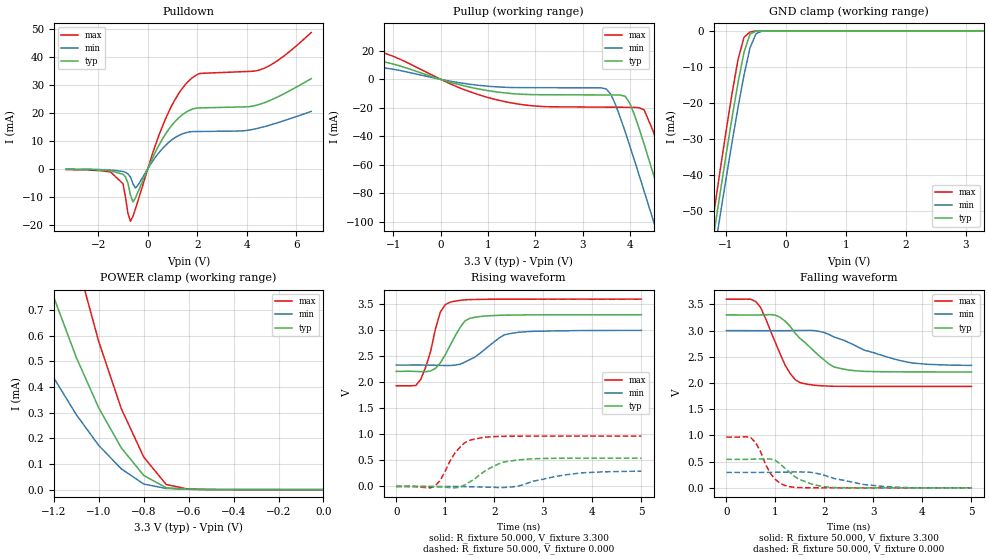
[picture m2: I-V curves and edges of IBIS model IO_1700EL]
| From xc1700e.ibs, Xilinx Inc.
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|   Model IO_1700EL
[Model]   IO_1700EL
Model_type   I/O
Polarity   Non-Inverting
Enable   Active-High
Vinl =   0.800V
Vinh =   2.000V
Vmeas =   1.650V
Cref =  50.000pF
Rref =   1.000M
Vref =  0.000V
C_comp   2.500pF   2.000pF   3.000pF
[Temperature Range]   50.000   100.000   0.000
[Voltage Range]   3.300V   3.000V   3.600V
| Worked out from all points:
|   slope of the pulldown table from 0 to 0.495 V, typ, clamps not added: 54.3 ohm
|   slope of the pullup table from 0 to 0.495 V, typ, clamps not added: 108 ohm
|   GND clamp passes 1 mA (typ) near -0.60 V on its own axis
|   POWER clamp passes 1 mA (typ) near -1.29 V on its own axis
|   rising waveform, R_fixture 50.000, V_fixture 3.300: 20-80 % time 389ps typ, 556ps min, 284ps max; typ from 2.21 V to 3.3 V
|   rising waveform, R_fixture 50.000, V_fixture 0.000: 20-80 % time 555ps typ, 874ps min, 383ps max; typ from 0 V to 0.543 V
|   falling waveform, R_fixture 50.000, V_fixture 3.300: 20-80 % time 706ps typ, 1.15ns min, 464ps max; typ from 3.3 V to 2.21 V
|   falling waveform, R_fixture 50.000, V_fixture 0.000: 20-80 % time 514ps typ, 842ps min, 321ps max; typ from 0.543 V to 0 V
[Pulldown]
| voltage   I(typ)   I(min)   I(max)
-3.3V     -200uA     -100uA     -300uA
-1.5V     -700uA     -440uA     -1.16mA
-1V       -1.96mA    -970uA     -5.37mA
-800mV    -5.18mA    -1.82mA    -15.96mA
-700mV    -9.413mA   -2.98mA    -18.75mA
-600mV    -11.79mA   -5.361mA   -17mA
-500mV    -10.41mA   -6.905mA   -14.34mA
600mV     10.73mA    7.28mA     15.37mA
1.6V      20.47mA    13.01mA    30.87mA
2.1V      21.72mA    13.3mA     34.02mA
4.7V      23.55mA    15.01mA    35.86mA
6.6V      32.17mA    20.46mA    48.6mA
[Pullup]
| voltage   I(typ)   I(min)   I(max)
-3.3V     22.13mA    12.6mA     35.43mA
-1.5V     14.78mA    9.662mA    22.26mA
1.2V      -8.899mA   -5.297mA   -14.5mA
3.5V      -10.96mA   -6.739mA   -19.54mA
3.7V      -10.99mA   -18.23mA   -19.58mA
4V        -16.93mA   -47.12mA   -19.65mA
4.3V      -45.58mA   -78.7mA    -21.49mA
4.5V      -67.23mA   -100mA     -37.14mA
4.7V      -89.56mA   -122mA     -58.71mA
4.9V      -112mA     -144mA     -81.58mA
5.1V      -135mA     -167mA     -105mA
6.6V      -313mA     -337mA     -289mA
[GND_clamp]
| voltage   I(typ)   I(min)   I(max)
-3.3V     -301mA     -296mA     -307mA
-1.3V     -67.23mA   -72.67mA   -61.75mA
-1.2V     -56.13mA   -62mA      -50.22mA
-1.1V     -45.21mA   -51.47mA   -38.91mA
-1V       -34.51mA   -41.11mA   -27.9mA
-900mV    -24.15mA   -31mA      -17.39mA
-800mV    -14.38mA   -21.28mA   -7.958mA
-700mV    -5.907mA   -12.25mA   -1.783mA
-600mV    -925uA     -4.729mA   -328uA
-500mV    -63.77uA   -772uA     -21.5uA
-400mV    -3.027uA   -71.54uA   -1.321uA
3.3V      152pA      11.15nA    59.2pA
[POWER_clamp]
| voltage   I(typ)   I(min)   I(max)
-3.3V     9.547mA    5.776mA    15.34mA
-1.4V     1.31mA     780uA      2.172mA
-1.3V     1.015mA    598uA      1.703mA
-1.2V     749uA      435uA      1.276mA
-1.1V     515uA      292uA      898uA
-1V       318uA      172uA      576uA
-900mV    163uA      81.04uA    316uA
-800mV    55.24uA    21.71uA    127uA
-700mV    7.221uA    4.5uA      19.75uA
-600mV    1.258uA    1.103uA    1.726uA
0V        152pA      1.498nA    69.06pA
[Ramp]
| variable   typ   min   max
dV/dt_r   0.326/0.560n   0.175/0.857n   0.581/0.376n
dV/dt_f   0.653/0.707n   0.398/1.106n   0.999/0.456n
R_load = 50.000
[Rising Waveform]
R_fixture = 50.000
V_fixture = 3.300
V_fixture_min = 3.000
V_fixture_max = 3.600
L_fixture = 0.000H
C_fixture = 0.000F
| time   V(typ)   V(min)   V(max)
0s        2.212V     2.333V     1.935V
400ps     2.21V      2.334V     1.94V
500ps     2.206V     2.334V     2.056V
700ps     2.218V     2.332V     2.589V
900ps     2.375V     2.327V     3.35V
1.1ns     2.711V     2.324V     3.541V
1.4ns     3.179V     2.389V     3.586V
1.6ns     3.251V     2.483V     3.593V
2.3ns     3.293V     2.934V     3.599V
5ns       3.3V       2.999V     3.6V
[Rising Waveform]
R_fixture = 50.000
V_fixture = 0.000
V_fixture_min = 0.000
V_fixture_max = 0.000
L_fixture = 0.000H
C_fixture = 0.000F
| time   V(typ)   V(min)   V(max)
0s        0V         0V         0V
800ps     -6.525mV   342uV      15.63mV
900ps     -11.2mV    389uV      121mV
1.3ns     -14.17mV   -2.964mV   753mV
1.5ns     87.7mV     -7.401mV   888mV
1.7ns     222mV      -10.74mV   930mV
2.1ns     438mV      -22.16mV   962mV
2.5ns     510mV      10.54mV    966mV
3.7ns     543mV      252mV      968mV
5ns       543mV      292mV      968mV
[Falling Waveform]
R_fixture = 50.000
V_fixture = 3.300
V_fixture_min = 3.000
V_fixture_max = 3.600
L_fixture = 0.000H
C_fixture = 0.000F
| time   V(typ)   V(min)   V(max)
0s        3.3V       3V         3.6V
600ps     3.299V     2.999V     3.555V
700ps     3.3V       2.999V     3.441V
1.1ns     3.253V     2.999V     2.55V
1.3ns     3.085V     3V         2.184V
1.5ns     2.852V     3.003V     2.01V
2.1ns     2.359V     2.924V     1.941V
2.4ns     2.264V     2.814V     1.937V
3.7ns     2.213V     2.398V     1.935V
5ns       2.212V     2.337V     1.935V
[Falling Waveform]
R_fixture = 50.000
V_fixture = 0.000
V_fixture_min = 0.000
V_fixture_max = 0.000
L_fixture = 0.000H
C_fixture = 0.000F
| time   V(typ)   V(min)   V(max)
0s        543mV      295mV      968mV
500ps     546mV      295mV      957mV
600ps     549mV      295mV      860mV
900ps     550mV      296mV      274mV
1.1ns     456mV      299mV      85.44mV
1.3ns     292mV      302mV      20.5mV
1.7ns     86.21mV    299mV      1.821mV
2.1ns     12.98mV    209mV      343uV
3.2ns     260uV      27.7mV     43.17uV
5ns       20.16uV    350uV      15.1uV
